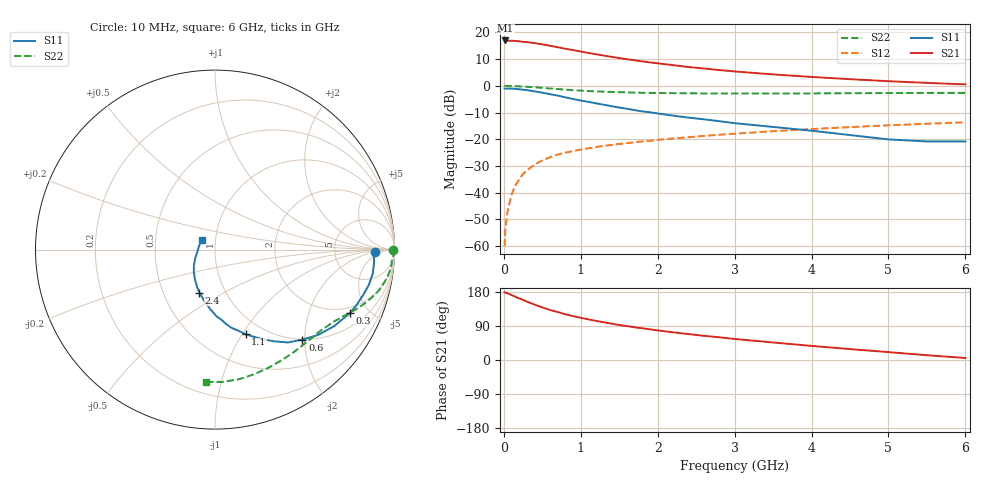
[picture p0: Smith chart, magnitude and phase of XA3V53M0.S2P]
! SIEMENS Discrete & RF Semiconductors
! BFY180
! Si NPN RF Bipolar Junction Transistor in MICRO-X
! VCE = 3.5 V  IC = 3 mA
! Common Emitter S-Parameters:  May  1997
# GHz  S  MA  R  50
!  f  S11  S21  S12  S22
! GHz  MAG  ANG  MAG  ANG  MAG  ANG  MAG  ANG
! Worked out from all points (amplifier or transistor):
!   36 points, 10 MHz to 6 GHz, reference 50 ohm
!   highest |S21| = 17.0 dB at 20 MHz (marker M1)
!   |S21| within 3 dB of that: start of sweep to 779.4 MHz
!   unconditionally stable (mu >= 1): 2.239 GHz to end of sweep
!   at 250 MHz: K = 0.18, MSG = 24.7 dB, |S12| = -33.0 dB
!   at 1.4 GHz: K = 0.81, MSG = 16.5 dB, |S12| = -22.1 dB
!   at 6 GHz: K = 1.07, MAG = 5.5 dB, |S12| = -13.7 dB
!   S11 on the Smith chart (normalised r, x): 10 MHz: 17, -2; 300 MHz: 1.66, -3.81; 600 MHz: 1.00, -1.95; 1.1 GHz: 0.82, -1.04; 2.4 GHz: 0.75, -0.39; 6 GHz: 0.86, +0.09
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0.01  0.8901 -0.9  7.011 178.7  0.001 79.0  0.993 -0.2
0.02  0.8859 -1.8  7.073 177.9  0.0022 90.9  0.9999 -0.7
0.05  0.8891 -4.5  6.993 175.6  0.0046 86.5  0.9936 -1.9
0.1  0.8892 -8.6  6.991 171.3  0.0092 85.6  0.987 -3.8
0.2  0.8636 -17.0  6.829 162.5  0.0177 79.8  0.9786 -7.6
0.3  0.8316 -25.1  6.585 154.1  0.0261 75.8  0.9603 -11.0
0.4  0.789 -32.7  6.303 146.1  0.0339 71.4  0.9403 -14.1
0.5  0.7454 -39.7  5.984 138.8  0.04 67.5  0.915 -16.8
0.6  0.6988 -45.8  5.63 131.9  0.0461 64.6  0.8922 -19.2
0.8  0.6088 -57.1  4.938 120.7  0.0563 59.3  0.8498 -23.2
1  0.5316 -66.0  4.39 111.2  0.0644 55.6  0.8145 -26.6
1.1  0.5015 -70.1  4.126 107.2  0.0678 54.4  0.8003 -27.9
1.3  0.4433 -78.4  3.678 99.6  0.0754 52.2  0.7776 -30.7
1.5  0.3926 -84.7  3.32 92.4  0.0818 50.4  0.7611 -33.5
1.7  0.3513 -91.5  3.017 86.3  0.0881 49.2  0.7464 -36.0
2.2  0.2772 -104.6  2.442 73.0  0.1036 45.7  0.7303 -42.5
2.4  0.2546 -110.1  2.25 68.4  0.1093 44.5  0.725 -45.1
3  0.2006 -123.9  1.861 55.5  0.1273 40.8  0.7203 -52.7
3.5  0.1702 -133.9  1.638 46.2  0.1416 37.6  0.7197 -59.1
4.5  0.12 -156.6  1.333 28.8  0.1691 30.5  0.7277 -72.4
5.5  0.0912 167.3  1.136 12.6  0.1955 22.8  0.7383 -86.6
6  0.0912 143.4  1.065 5.3  0.2076 18.5  0.739 -93.7
